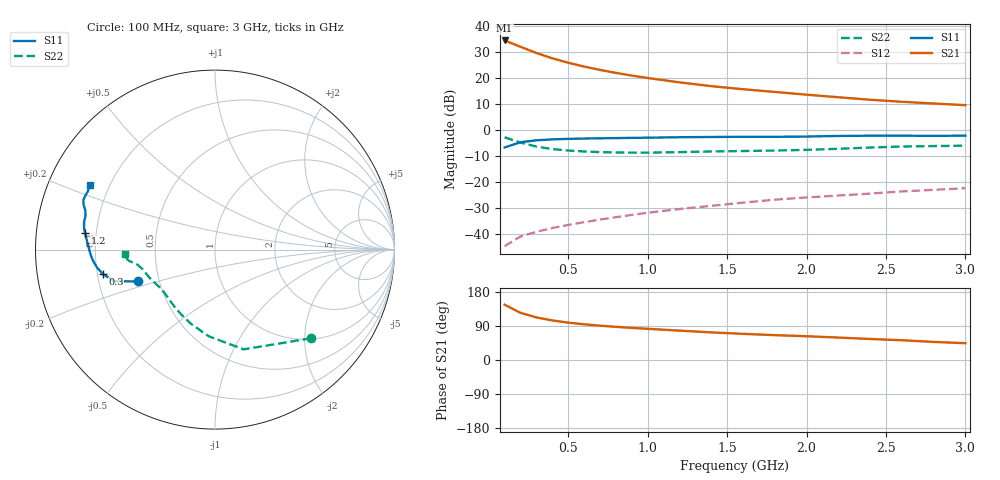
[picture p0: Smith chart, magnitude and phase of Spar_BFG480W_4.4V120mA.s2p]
! Filename: 4_4120BFG480.001
! Title: BFG480W
! Bias: Vce=4.4V; Ic=120mA
! Company: NXP Semiconductors NL
! User: Quality&Reliability T&D
! Measure time: 10 Nov 1999 / 12:07:28
#  MHz  S  MA  R 50
! Freq  S11  S21  S12  S22  :
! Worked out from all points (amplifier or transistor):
!   20 points, 100 MHz to 3 GHz, reference 50 ohm
!   highest |S21| = 34.4 dB at 100 MHz (marker M1)
!   |S21| within 3 dB of that: start of sweep to 224.1 MHz
!   unconditionally stable (mu >= 1): 646.4 MHz to end of sweep
!   at 400 MHz: K = 0.85, MSG = 32.6 dB, |S12| = -37.5 dB
!   at 1.2 GHz: K = 1.09, MAG = 22.5 dB, |S12| = -30.3 dB
!   at 3 GHz: K = 1.05, MAG = 14.6 dB, |S12| = -22.3 dB
!   S11 on the Smith chart (normalised r, x): 100 MHz: 0.38, -0.17; 300 MHz: 0.22, -0.10; 1.2 GHz: 0.16, +0.06; 3 GHz: 0.13, +0.24
100  0.4657 -157.6  52.54 145.8  0.00596 68.1  0.7289 -42.6
200  0.5871 -162.5  39.73 124.5  0.009139 60.6  0.5783 -74.0
300  0.6393 -167.7  30.22 112.4  0.01125 60.3  0.4842 -94.2
400  0.6657 -171.5  23.92 104.4  0.01327 62.4  0.4343 -108.0
500  0.6811 -174.5  19.66 98.6  0.01522 64.8  0.4064 -118.0
600  0.6909 -176.9  16.58 94.2  0.0172 66.5  0.3902 -125.3
700  0.6978 -179.1  14.32 90.6  0.01926 68.8  0.3796 -131.0
800  0.704 179.0  12.55 87.5  0.02141 70.4  0.3734 -135.8
900  0.7115 177.1  11.14 84.8  0.0237 72.2  0.3705 -139.9
1000  0.7175 175.4  10.02 82.3  0.02609 73.1  0.3709 -143.5
1200  0.7317 172.6  8.263 77.5  0.03071 74.6  0.3792 -149.5
1400  0.7402 170.3  6.992 72.9  0.03535 75.5  0.3906 -153.9
1600  0.7458 167.9  6.096 69.0  0.04076 76.2  0.3981 -157.2
1800  0.7454 165.4  5.416 65.6  0.04639 76.7  0.4066 -160.9
2000  0.7546 163.2  4.794 62.7  0.05122 77.1  0.4193 -165.2
2200  0.774 161.1  4.278 59.2  0.05581 77.1  0.4394 -168.9
2400  0.7837 159.3  3.833 55.5  0.06072 76.5  0.4646 -171.2
2600  0.7831 157.7  3.502 52.1  0.0669 75.7  0.4853 -172.7
2800  0.7791 155.4  3.247 47.7  0.07167 74.3  0.4957 -174.4
3000  0.7839 152.8  3.015 44.3  0.07706 73.5  0.504 -177.3
